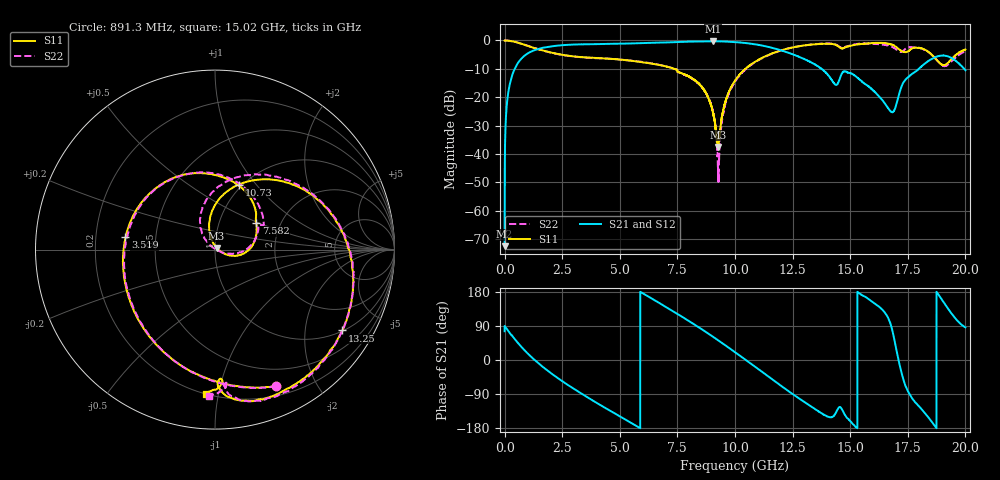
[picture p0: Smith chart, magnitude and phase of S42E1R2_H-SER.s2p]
! Created Wed Nov 25 21:32:29 2020
# khz S ma R 50
! 2 Port Network Data from SP1.SP block
! freq  magS11  angS11  magS21  angS21  magS12  angS12  magS22  angS22
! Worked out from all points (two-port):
!   20001 points, 300 kHz to 20 GHz, reference 50 ohm
!   highest |S21| = -0.28 dB at 9.043 GHz (marker M1); lowest = -72.4 dB at 300 kHz (marker M2)
!   |S21| within 3 dB of the highest: 1.352 GHz to 11.92 GHz (10.56 GHz wide, 159 % of centre); 11.91848 GHz to 11.91951 GHz (1.021 MHz wide, 0.00857 % of centre)
!   lowest |S11| = -37.5 dB at 9.266 GHz (marker M3), VSWR 1.03, Z = 50.9 + j0.994 ohm
!   |S11| at or under -10 dB: 7.361994 GHz to 7.363525 GHz (1.531 MHz wide, 0.0208 % of centre); 7.364991 GHz to 7.366585 GHz (1.593 MHz wide, 0.0216 % of centre); 7.368 GHz to 10.45 GHz (3.079 GHz wide, 34.6 % of centre)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
!   |S22| runs from -50.2 to 0.0 dB; largest |S21 - S12| = 0.011
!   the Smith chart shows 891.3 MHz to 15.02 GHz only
!   S11 on the Smith chart (normalised r, x): 891.3 MHz: 0.30, -1.50; 3.519 GHz: 0.33, +0.06; 7.582 GHz: 1.50, +0.48; 10.73 GHz: 0.96, +0.82; 13.25 GHz: 1.02, -3.14; 15.02 GHz: 0.20, -0.92
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300  0.9936 -0.2  0.0002394 75.9  0.0002196 92.4  0.9963 -0.2
103300  0.9964 -8.4  0.07923 81.4  0.07958 81.3  0.9959 -8.3
181300  0.9894 -14.8  0.1378 74.8  0.1386 74.7  0.9885 -14.6
891300  0.8331 -66.0  0.5495 24.1  0.5486 24.1  0.8353 -65.8
1880300  0.6327 -118.3  0.7714 -28.7  0.7729 -28.8  0.6288 -118.9
3334300  0.5091 179.4  0.8544 -88.6  0.8537 -88.6  0.5063 -176.4
3519300  0.5036 172.2  0.8561 -95.5  0.8564 -95.6  0.4991 176.9
5223300  0.4537 113.4  0.8812 -156.5  0.8828 -156.5  0.4532 114.6
6667300  0.3735 66.0  0.9164 152.1  0.9139 152.1  0.3755 60.5
7582300  0.2732 32.9  0.9428 118.7  0.9424 118.9  0.2713 27.2
9043300  0.05454 -23.1  0.9687 61.4  0.9673 61.3  0.05548 -19.2
9266300  0.01328 47.3  0.9642 52.1  0.9667 52.0  0.004137 17.2
1.00003e7  0.1956 96.7  0.9367 20.5  0.9363 20.6  0.187 116.5
1.07313e7  0.3862 69.8  0.8715 -11.6  0.8687 -11.3  0.3816 81.0
1.19073e7  0.6523 22.9  0.6882 -63.9  0.6886 -63.7  0.6481 24.5
1.32503e7  0.8403 -32.4  0.4237 -120.5  0.4237 -120.6  0.84 -32.2
1.33343e7  0.8461 -36.1  0.4052 -124.0  0.4085 -124.2  0.8477 -35.5
1.50233e7  0.8056 -93.8  0.264 -162.5  0.2636 -162.6  0.8162 -92.5
1.66673e7  0.8753 -154.1  0.06277 108.5  0.06163 109.7  0.8135 -159.5
1.80413e7  0.732 163.0  0.3349 -125.6  0.3377 -125.2  0.7328 163.7
1.88453e7  0.4124 135.7  0.5324 171.2  0.5308 171.3  0.4125 141.5
2e7  0.6948 139.1  0.2998 86.1  0.3008 87.0  0.6383 139.7
